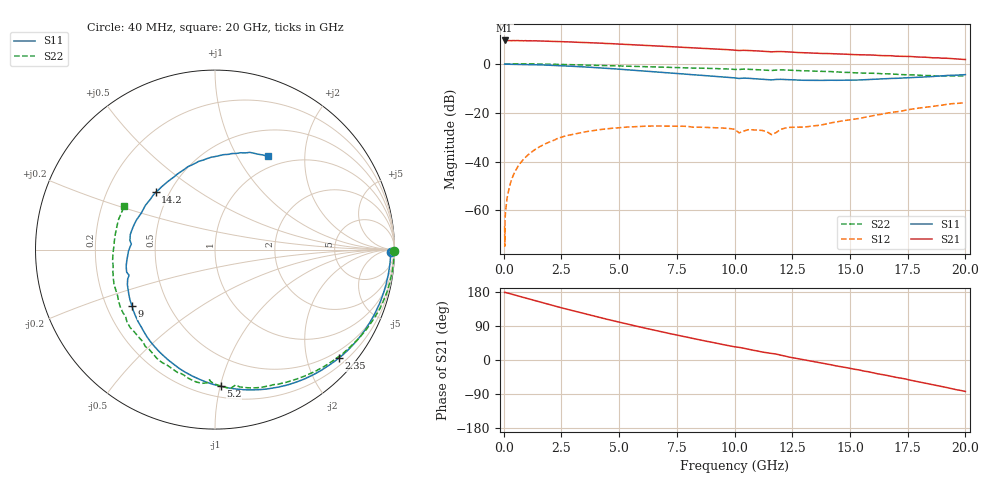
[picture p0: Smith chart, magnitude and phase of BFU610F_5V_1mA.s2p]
! Filename:  P:\Prog\Test\Noise\ATS_data\Testdata_Net\SplitFiles\BFU610_2W_A5_HighFreq_5V_1mA_D.s2p
! Date/Time: Wed 10/Aug/2011 16:58:05
! BFU610_2W_A5_HighFreq_5V_1mA_10mA_Bias1_R.s2p
! MDIF S-parameter v. bias file
! BFU610_2W_A5_HighFreq_5V_1mA_10mA
! Date/time Mon Aug 08 14:15:19 2011
! bias mode 1
! bias variable = I_out
! VAR bias_var= 1
! VAR V_out= 5.0010
! VAR I_out= 0.9950
! VAR V_in= 0.8432
! VAR I_in= 0.0064
! Device data file deembeded for feedlines and parallel
! Original file: \SplitFiles\BFU610_2W_A5_HighFreq_5V_1mA_R.s2p
! Feed-files: PR003V01_101208_Feed1.s2p, PR003V01_101208_Feed2.s2p
! Parallel-file: PR003V01_101208_Par.s2p
# MHz S MA R 50
!  Freq-MHz  S11-mag  S11-arg  S21-mag  S21-arg  S12-mag  S12-arg  S22-mag  S22-arg
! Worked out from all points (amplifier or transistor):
!   167 points, 40 MHz to 20 GHz, reference 50 ohm
!   highest |S21| = 9.5 dB at 40 MHz (marker M1)
!   |S21| within 3 dB of that: start of sweep to 8.162 GHz
!   unconditionally stable (mu >= 1): 7.942 GHz to end of sweep
!   at 550 MHz: K = 0.00, MSG = 26.3 dB, |S12| = -43.1 dB
!   at 4.2 GHz: K = 0.37, MSG = 17.7 dB, |S12| = -26.9 dB
!   at 20 GHz: K = 1.03, MAG = 7.7 dB, |S12| = -15.9 dB
!   S11 on the Smith chart (normalised r, x): 40 MHz: 70, -40; 2.35 GHz: 0.34, -2.62; 5.2 GHz: 0.28, -1.00; 9 GHz: 0.31, -0.28; 14.2 GHz: 0.42, +0.34; 20 GHz: 0.84, +1.36
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40  0.9787 -0.7  2.993 178.7  0.0004787 76.0  0.9974 -0.3
50  0.9705 -1.1  2.98 179.0  0.0001857 84.4  0.9976 -0.5
60  0.9792 -0.8  2.982 178.1  0.0006511 98.9  0.9983 -0.5
140  0.9785 -2.5  2.974 177.3  0.001681 88.2  0.998 -1.3
320  0.977 -5.7  2.957 174.3  0.003963 88.2  0.998 -3.0
600  0.9731 -10.7  2.981 169.5  0.007692 85.2  0.996 -5.7
1250  0.959 -22.1  2.93 158.4  0.01618 76.5  0.9891 -11.8
2350  0.9171 -41.2  2.853 140.2  0.03004 63.3  0.9687 -22.0
3400  0.8656 -58.7  2.725 123.7  0.03936 49.5  0.9435 -31.2
4300  0.8155 -73.3  2.623 110.1  0.04572 39.9  0.9196 -38.5
5200  0.7623 -87.6  2.495 97.1  0.05015 31.2  0.8949 -45.6
6800  0.6695 -112.5  2.287 75.0  0.05316 17.7  0.8526 -57.8
9000  0.5592 -145.8  2.027 47.1  0.04947 7.6  0.8016 -73.9
10200  0.4996 -163.4  1.863 33.3  0.03852 1.4  0.7628 -81.3
10800  0.4959 -172.6  1.847 25.9  0.04448 9.8  0.761 -87.2
11600  0.4672 176.3  1.753 17.3  0.03545 12.2  0.7257 -92.4
12000  0.4795 170.0  1.774 12.8  0.04554 26.9  0.7491 -95.6
13400  0.4595 147.6  1.649 -3.9  0.05366 24.8  0.7064 -109.3
14200  0.4598 135.9  1.606 -12.9  0.06211 28.0  0.6901 -117.3
16800  0.5007 100.1  1.458 -43.2  0.101 20.5  0.6169 -148.8
18400  0.5432 80.1  1.346 -63.0  0.1311 8.0  0.5732 -174.3
20000  0.5984 60.1  1.218 -83.0  0.1595 -8.7  0.56 154.4
